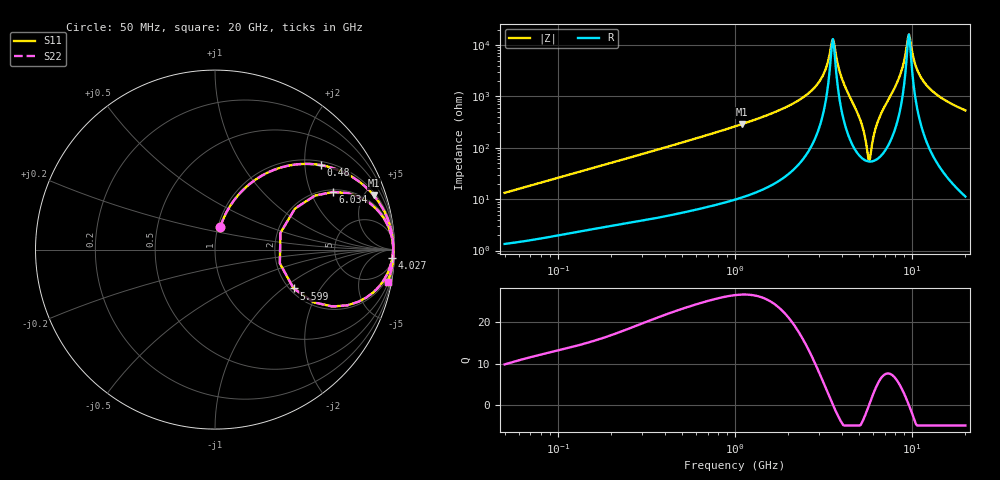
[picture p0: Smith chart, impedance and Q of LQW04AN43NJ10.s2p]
!Murata Part Number: LQW04AN43NJ10
!These Parameters are Measured in Series Mode Connection
!  o--[Z]--o
!Port1  Port2
!  o-------o
!Freq. Start=50[MHz] Stop=20[GHz], 401[Steps]
# Hz S RI R 50
!Freq.(Hz) S11(Real) S11(Imag) S21(Real) S21(Imag) S12(Real) S12(Imag) S22(Real) S22(Imag)
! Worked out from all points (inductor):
!   401 points, 50 MHz to 20 GHz, reference 50 ohm
!   read as one part in series: L = 41.8 nH near 51.52 MHz
!   highest Q = 26.8 at 1.094 GHz (marker M1), where L = 42 nH
!   self-resonance near 3.519 GHz
!   S11 on the Smith chart (normalised r, x): 50 MHz: 1.03, +0.26; 480 MHz: 1.11, +2.42; 4.027 GHz: 10, -42; 5.599 GHz: 2.10, -1.19; 6.034 GHz: 2.10, +2.92; 20 GHz: 1, -11
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5e7  0.0298 0.1265  0.9702 -0.1265  0.9702 -0.1265  0.0298 0.1265
1.364002e8  0.1261 0.2996  0.8739 -0.2996  0.8739 -0.2996  0.1261 0.2996
3.721004e8  0.4697 0.4762  0.5303 -0.4762  0.5303 -0.4762  0.4697 0.4762
4.800071e8  0.5905 0.4705  0.4095 -0.4705  0.4095 -0.4705  0.5905 0.4705
1e9  0.8628 0.3258  0.1372 -0.3258  0.1372 -0.3258  0.8628 0.3258
1.094034e9  0.884 0.302  0.116 -0.302  0.116 -0.302  0.884 0.302
2.728004e9  0.9882 0.0733  0.0118 -0.0733  0.0118 -0.0733  0.9882 0.0733
3.168813e9  0.9921 0.035  0.00793 -0.035  0.00793 -0.035  0.9921 0.035
3.572216e9  0.9924 -1.19e-05  0.00758 1.19e-05  0.00758 1.19e-05  0.9924 -1.19e-05
4.026975e9  0.9882 -0.044  0.0118 0.044  0.0118 0.044  0.9882 -0.044
5.041459e9  0.901 -0.2198  0.099 0.2198  0.099 0.2198  0.901 -0.2198
5.352748e9  0.7375 -0.3105  0.2625 0.3105  0.2625 0.3105  0.7375 -0.3105
5.598765e9  0.4381 -0.2167  0.5619 0.2167  0.5619 0.2167  0.4381 -0.2167
5.769027e9  0.3646 0.0931  0.6354 -0.0931  0.6354 -0.0931  0.3646 0.0931
6.034176e9  0.6581 0.3215  0.3419 -0.3215  0.3419 -0.3215  0.6581 0.3215
6.503449e9  0.8981 0.2274  0.1019 -0.2274  0.1019 -0.2274  0.8981 0.2274
7.442007e9  0.9757 0.1016  0.0243 -0.1016  0.0243 -0.1016  0.9757 0.1016
8.516016e9  0.9905 0.0385  0.00952 -0.0385  0.00952 -0.0385  0.9905 0.0385
9.600142e9  0.9938 -0.000409  0.00616 0.000409  0.00616 0.000409  0.9938 -0.000409
1.066139e10  0.9938 -0.0289  0.00617 0.0289  0.00617 0.0289  0.9938 -0.0289
1.201863e10  0.9918 -0.0585  0.00821 0.0585  0.00821 0.0585  0.9918 -0.0585
2e10  0.9628 -0.1791  0.0372 0.1791  0.0372 0.1791  0.9628 -0.1791
